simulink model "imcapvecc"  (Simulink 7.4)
settings: Solver=ode45  StartTime=0  StopTime=15  MaxStep=5e-4  RelTol=1e-4
libraries: simulink x2

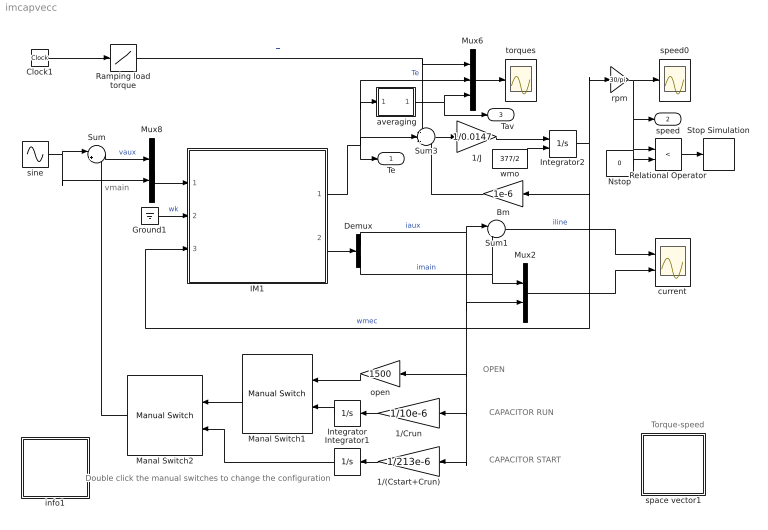
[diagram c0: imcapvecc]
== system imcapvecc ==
  note: OPEN
  note: CAPACITOR RUN
  note: CAPACITOR START
  note: vmain
  note: Torque-speed
  note: Double click the manual switches to change the configuration
  " averaging" : Subsystem
  1/(Cstart+Crun) : Gain  Gain=1/213e-6  ParameterDataType=sfix(16)  ParameterScaling=2^0  OutDataType=sfix(16)  OutScaling=2^0
  1/Crun : Gain  Gain=1/10e-6  ParameterDataType=sfix(16)  ParameterScaling=2^0  OutDataType=sfix(16)  OutScaling=2^0
  1/J : Gain  Gain=1/0.0147  ParameterDataType=sfix(16)  ParameterScaling=2^0  OutDataType=sfix(16)  OutScaling=2^0
  Bm : Gain  Gain=1e-6  ParameterDataType=sfix(16)  ParameterScaling=2^0  OutDataType=sfix(16)  OutScaling=2^0
  Clock1 : Clock
  Demux : Demux  Outputs=2
  Ground1 : Ground
  IM1 : Subsystem  mask(Inductionmachine){Rs=2.02, Rr=4.12, Lsl=8.54e-3, Lrl=3.13e-3, Lm=180e-3, wo=2*pi*60, p=4}
      mask prompts: Rs "Stator resistance [ohm]"; Rr "Rotor resistance [ohm]"; Lsl "Stator leakage inductance  [H]"; Lrl "Rotor leakage inductance [H]"; Lm "Magnetizing inductance [H]"; wo "Base frequency [rad/s]"; p "Number of poles"
      mask help: Space vector model of the induction machine in a general frame k. SI units
  Integrator : Integrator
  Integrator1 : Integrator
  Integrator2 : Integrator  InitialConditionSource=external  InitialCondition=377/2
  Manal Switch1 : simulink/Signal Routing/Manual Switch  SystemSampleTime=-1  sw=1  action=0  varsize=off
  Manal Switch2 : simulink/Signal Routing/Manual Switch  SystemSampleTime=-1  sw=0  action=0  varsize=off
  Mux2 : Mux  Inputs=2
  Mux6 : Mux  Inputs=3
  Mux8 : Mux  Inputs=2
  Nstop : Constant  Value=0  OutDataType=sfix(16)  OutScaling=2^0
  Ramping load torque : Lookup  InputValues=[0 1 5]  Table=[0 0 3.50]  OutDataType=sfix(16)  OutScaling=2^0
  Relational Operator : RelationalOperator  Operator=<
  Stop Simulation : Stop
  Sum : Sum  Inputs=|+-  OutDataType=sfix(16)  OutScaling=2^0
  Sum1 : Sum  Inputs=|++  OutDataType=sfix(16)  OutScaling=2^0
  Sum3 : Sum  Inputs=-+-  OutDataType=sfix(16)  OutScaling=2^0
  current : Scope  NumInputPorts=2
  info1 : Subsystem
  open : Gain  Gain=1500  ParameterDataType=sfix(16)  ParameterScaling=2^0  OutDataType=sfix(16)  OutScaling=2^0
  rpm : Gain  Gain=30/pi  ParameterDataType=sfix(16)  ParameterScaling=2^0  OutDataType=sfix(16)  OutScaling=2^0
  sine : Sin  Amplitude=110*sqrt(2)  Bias=0  Frequency=2*pi*60  Phase=pi/2  Samples=10  SampleTime=0
  space vector1 : Subsystem
  speed0 : Scope
  torques : Scope
  wmo : Constant  Value=377/2  OutDataType=sfix(16)  OutScaling=2^0
  Te : Outport
  speed : Outport  Port=2
  Tav : Outport  Port=3
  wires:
  Sum1/1 -> current/1  "iline"
  Mux2/1 -> current/2
  Mux8/1 -> IM1/1(vs)
  Sum/1 -> Mux8/1  "vaux"
  sine/1 -> Mux8/2, Sum/1
  IM1/2(is) -> Demux/1
  Demux/1 -> Sum1/1, Mux2/2, open/1, 1/(Cstart+Crun)/1, 1/Crun/1  "iaux"
  Demux/2 -> Sum1/2, Mux2/1  "imain"
  1/J/1 -> Integrator2/1
  Mux6/1 -> torques/1
  Bm/1 -> Sum3/3
  Integrator2/1 -> Bm/1, IM1/3(wmec), rpm/1  "wmec"
  rpm/1 -> speed0/1, speed/1, Relational Operator/1
  IM1/1(Te) -> Sum3/2, Te/1, Mux6/2, " averaging"/1(sig)  "Te"
  Sum3/1 -> 1/J/1
  Clock1/1 -> Ramping load torque/1
  Ramping load torque/1 -> Mux6/1, Sum3/1  "Tl"
  Ground1/1 -> IM1/2(wk)  "wk"
  " averaging"/1(ave) -> Mux6/3, Tav/1
  open/1 -> Manal Switch1/1
  Integrator/1 -> Manal Switch1/2
  1/Crun/1 -> Integrator/1
  Manal Switch1/1 -> Manal Switch2/1
  Manal Switch2/1 -> Sum/2
  1/(Cstart+Crun)/1 -> Integrator1/1
  Integrator1/1 -> Manal Switch2/2
  wmo/1 -> Integrator2/2
  Nstop/1 -> Relational Operator/2
  Relational Operator/1 -> Stop Simulation/1

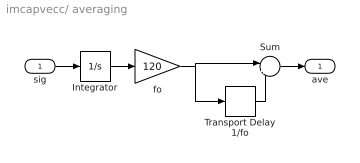
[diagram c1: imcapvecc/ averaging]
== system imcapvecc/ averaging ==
  sig : Inport  OutDataType=sfix(16)  OutScaling=2^0
  Integrator : Integrator
  Sum : Sum  Inputs=|+-  OutDataType=sfix(16)  OutScaling=2^0
  Transport Delay 1/fo : TransportDelay  DelayTime=1/120
  fo : Gain  Gain=120  ParameterDataType=sfix(16)  ParameterScaling=2^0  OutDataType=sfix(16)  OutScaling=2^0
  ave : Outport
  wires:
  Sum/1 -> ave/1
  Transport Delay 1/fo/1 -> Sum/2
  sig/1 -> Integrator/1
  fo/1 -> Transport Delay 1/fo/1, Sum/1
  Integrator/1 -> fo/1

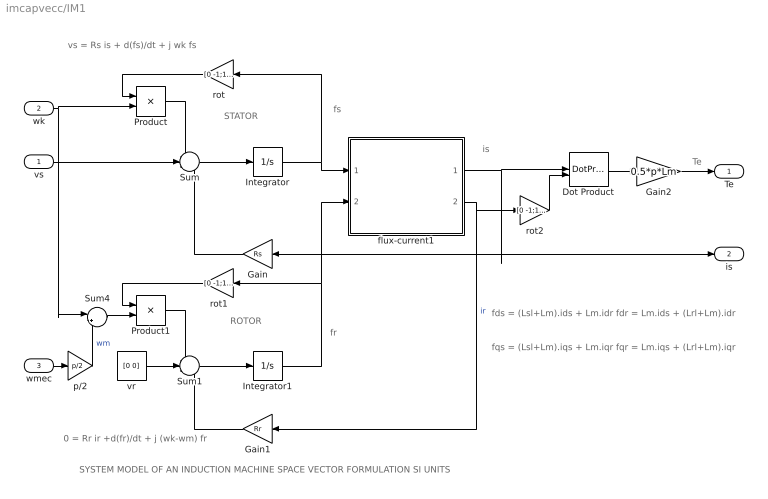
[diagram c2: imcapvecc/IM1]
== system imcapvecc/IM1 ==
  note: ROTOR
  note: STATOR
  note: fs
  note: is
  note: Te
  note: SYSTEM MODEL OF AN INDUCTION MACHINE SPACE VECTOR FORMULATION SI UNITS
  note: vs = Rs is + d(fs)/dt + j wk fs
  note: 0 = Rr ir +d(fr)/dt + j (wk-wm) fr
  note: fds = (Lsl+Lm).ids + Lm.idr fdr = Lm.ids + (Lrl+Lm).idr
  note: fqs = (Lsl+Lm).iqs + Lm.iqr fqr = Lm.iqs + (Lrl+Lm).iqr
  note: fr
  vs : Inport  OutDataType=sfix(16)  OutScaling=2^0
  wk : Inport  Port=2  OutDataType=sfix(16)  OutScaling=2^0
  wmec : Inport  Port=3  OutDataType=sfix(16)  OutScaling=2^0
  Dot Product : DotProduct  OutDataType=fixdt(1, 16)  OutScaling=2^-10
  Gain : Gain  Gain=Rs  ParameterDataType=sfix(16)  ParameterScaling=2^0  OutDataType=sfix(16)  OutScaling=2^0
  Gain1 : Gain  Gain=Rr  ParameterDataType=sfix(16)  ParameterScaling=2^0  OutDataType=sfix(16)  OutScaling=2^0
  Gain2 : Gain  Gain=0.5*p*Lm  ParameterDataType=sfix(16)  ParameterScaling=2^0  OutDataType=sfix(16)  OutScaling=2^0
  Integrator : Integrator  InitialCondition=[0 0]
  Integrator1 : Integrator  InitialCondition=[0 0]
  Product : Product  OutDataType=sfix(16)  OutScaling=2^0
  Product1 : Product  OutDataType=sfix(16)  OutScaling=2^0
  Sum : Sum  Inputs=-+-  OutDataType=sfix(16)  OutScaling=2^0
  Sum1 : Sum  Inputs=-+-  OutDataType=sfix(16)  OutScaling=2^0
  Sum4 : Sum  Inputs=|+-  OutDataType=sfix(16)  OutScaling=2^0
  flux-current1 : Subsystem
  p/2 : Gain  Gain=p/2  ParameterDataType=sfix(16)  ParameterScaling=2^0  OutDataType=sfix(16)  OutScaling=2^0
  rot : Gain  Gain=[0 -1;1 0]  Multiplication=Matrix(K*u)  ParameterDataType=sfix(16)  ParameterScaling=2^0  OutDataType=sfix(16)  OutScaling=2^0
  rot1 : Gain  Gain=[0 -1;1 0]  Multiplication=Matrix(K*u)  ParameterDataType=sfix(16)  ParameterScaling=2^0  OutDataType=sfix(16)  OutScaling=2^0
  rot2 : Gain  Gain=[0 -1;1 0]  Multiplication=Matrix(K*u)  ParameterDataType=sfix(16)  ParameterScaling=2^0  OutDataType=sfix(16)  OutScaling=2^0
  vr : Constant  Value=[0 0]  OutDataType=sfix(16)  OutScaling=2^0
  Te : Outport
  is : Outport  Port=2
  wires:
  Gain/1 -> Sum/3
  vr/1 -> Sum1/2
  Gain1/1 -> Sum1/3
  Integrator/1 -> flux-current1/1(fs), rot/1
  Integrator1/1 -> rot1/1, flux-current1/2(fr)
  Product1/1 -> Sum1/1
  rot1/1 -> Product1/1
  Product/1 -> Sum/1
  rot/1 -> Product/1
  Sum4/1 -> Product1/2
  vs/1 -> Sum/2
  wk/1 -> Product/2, Sum4/1
  Sum1/1 -> Integrator1/1
  Sum/1 -> Integrator/1
  flux-current1/1(is) -> Gain/1, is/1, Dot Product/1
  Dot Product/1 -> Gain2/1
  Gain2/1 -> Te/1
  wmec/1 -> p/2/1
  p/2/1 -> Sum4/2  "wm"
  rot2/1 -> Dot Product/2
  flux-current1/2(ir) -> Gain1/1, rot2/1  "ir"

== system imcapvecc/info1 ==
  note: Three configurations can be studied: A) Single phase B) Capacitor run C) Capacitor start
  note: Quasi-static characteristics of a single-phase capacitor induction motor:
  note: Compare the torque-speed curves with those derived from steady-state analysis. Select run capacitance such that the 120-Hertz torque pulsations are minimized at a specified speed.

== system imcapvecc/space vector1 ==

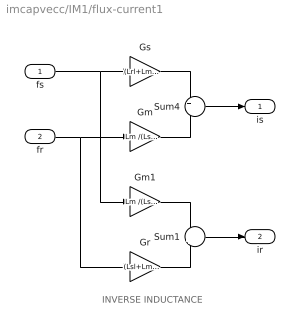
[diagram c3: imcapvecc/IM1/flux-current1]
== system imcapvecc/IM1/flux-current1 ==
  note: INVERSE INDUCTANCE
  fs : Inport  OutDataType=sfix(16)  OutScaling=2^0
  fr : Inport  Port=2  OutDataType=sfix(16)  OutScaling=2^0
  Gm : Gain  Gain=Lm /(Lsl*Lrl+Lsl*Lm+Lrl*Lm)  ParameterDataType=sfix(16)  ParameterScaling=2^0  OutDataType=sfix(16)  OutScaling=2^0
  Gm1 : Gain  Gain=Lm /(Lsl*Lrl+Lsl*Lm+Lrl*Lm)  ParameterDataType=sfix(16)  ParameterScaling=2^0  OutDataType=sfix(16)  OutScaling=2^0
  Gr : Gain  Gain=(Lsl+Lm )/(Lsl*Lrl+Lsl*Lm+Lrl*Lm)  ParameterDataType=sfix(16)  ParameterScaling=2^0  OutDataType=sfix(16)  OutScaling=2^0
  Gs : Gain  Gain=(Lrl+Lm) /(Lsl*Lrl+Lsl*Lm+Lrl*Lm)  ParameterDataType=sfix(16)  ParameterScaling=2^0  OutDataType=sfix(16)  OutScaling=2^0
  Sum1 : Sum  Inputs=-+  OutDataType=sfix(16)  OutScaling=2^0
  Sum4 : Sum  Inputs=+-  OutDataType=sfix(16)  OutScaling=2^0
  is : Outport
  ir : Outport  Port=2
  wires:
  fs/1 -> Gs/1, Gm1/1
  Gs/1 -> Sum4/1
  fr/1 -> Gm/1, Gr/1
  Gm/1 -> Sum4/2
  Sum4/1 -> is/1
  Gm1/1 -> Sum1/1
  Gr/1 -> Sum1/2
  Sum1/1 -> ir/1
